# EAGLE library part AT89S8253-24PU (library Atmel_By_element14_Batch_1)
MCU
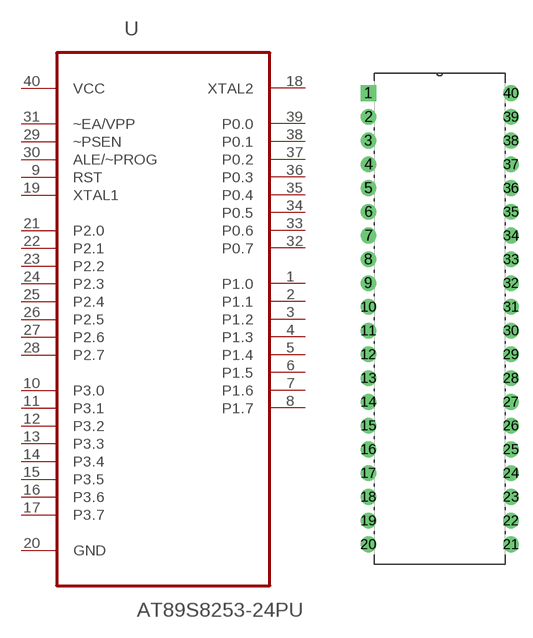
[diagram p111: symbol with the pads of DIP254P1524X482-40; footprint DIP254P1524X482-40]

Designator prefix U

## AT89S8253-24PU (DESCRIPTION: MCU; MPN: AT89S8253-24PU; OC_FARNELL: 1095746; OC_NEWARK: 96K6582; PACKAGE: DIP-40; SUPPLIER: Atmel)  [DIP254P1524X482-40]
1  P1.0
2  P1.1
3  P1.2
4  P1.3
5  P1.4
6  P1.5
7  P1.6
8  P1.7
9  RST  in
10  P3.0
11  P3.1
12  P3.2
13  P3.3
14  P3.4
15  P3.5
16  P3.6
17  P3.7
18  XTAL2  out
19  XTAL1  in
20  GND  pas
21  P2.0
22  P2.1
23  P2.2
24  P2.3
25  P2.4
26  P2.5
27  P2.6
28  P2.7
29  ~PSEN  in
30  ALE/~PROG  in
31  ~EA/VPP  in
32  P0.7
33  P0.6
34  P0.5
35  P0.4
36  P0.3
37  P0.2
38  P0.1
39  P0.0
40  VCC  pwr

## Footprint DIP254P1524X482-40 (pad centres in mm)
drill 1.118 square: 1 -15.24,48.26
drill 1.118: 2 -15.24,45.72; 3 -15.24,43.18; 4 -15.24,40.64; 5 -15.24,38.1; 6 -15.24,35.56; 7 -15.24,33.02; 8 -15.24,30.48; 9 -15.24,27.94; 10 -15.24,25.4; 11 -15.24,22.86; 12 -15.24,20.32; 13 -15.24,17.78; 14 -15.24,15.24; 15 -15.24,12.7; 16 -15.24,10.16; 17 -15.24,7.62; 18 -15.24,5.08; 19 -15.24,2.54; 20 -15.24,0; 21 0,0; 22 0,2.54; 23 0,5.08; 24 0,7.62; 25 0,10.16; 26 0,12.7; 27 0,15.24; 28 0,17.78; 29 0,20.32; 30 0,22.86; 31 0,25.4; 32 0,27.94; 33 0,30.48; 34 0,33.02; 35 0,35.56; 36 0,38.1; 37 0,40.64; 38 0,43.18; 39 0,45.72; 40 0,48.26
